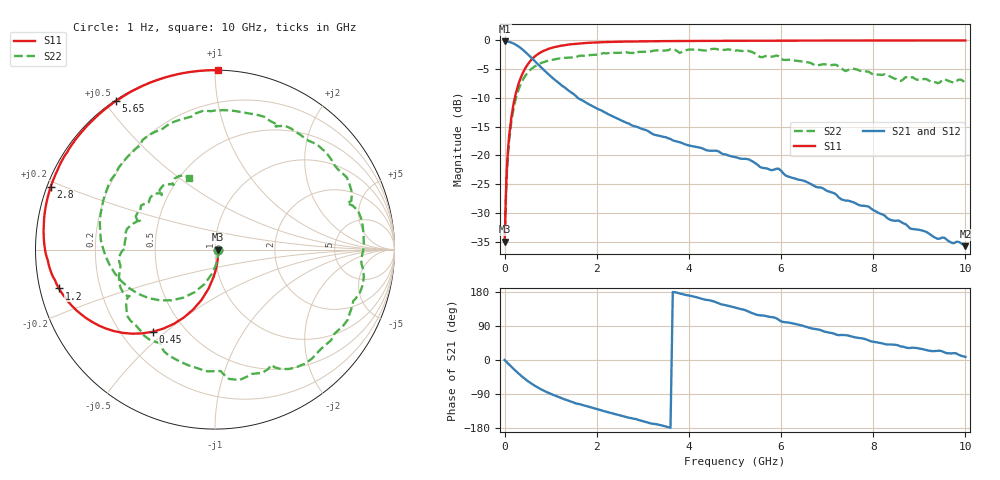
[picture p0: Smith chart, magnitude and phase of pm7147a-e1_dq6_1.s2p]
# GHz S DB R 50
! S-Parameters data
! Freq  dbS11  angS11  dbS21  angS21  dbS12  angS12  dbS22  angS22
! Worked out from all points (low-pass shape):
!   279 points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, 1 Hz to 10 GHz, reference 50 ohm
!   highest |S21| = -0.16 dB at 316.2 Hz (marker M1); lowest = -35.8 dB at 10 GHz (marker M2)
!   |S21| within 3 dB of the highest: start of sweep to 599.2 MHz
!   lowest |S11| = -35.0 dB at 316.2 Hz (marker M3), VSWR 1.04, Z = 51.8 - j4.22e-05 ohm
!   |S11| at or under -10 dB: start of sweep to 221.7 MHz
!   |S22| runs from -35.0 to -1.4 dB; largest |S21 - S12| = 3.9e-14
!   S11 on the Smith chart (normalised r, x): 1 Hz: 1.04, -0.00; 450 MHz: 0.33, -0.45; 1.2 GHz: 0.06, -0.12; 2.8 GHz: 0.01, +0.18; 5.65 GHz: 0.00, +0.54; 10 GHz: 0.00, +1.02
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1e-09  -35.00 -0.0  -0.16 -0.0  -0.16 -0.0  -35.00 -0.0
3.162e-07  -35.00 -0.0  -0.16 -0.0  -0.16 -0.0  -35.00 -0.0
0.03162278  -25.91 -71.9  -0.17 -3.9  -0.17 -3.9  -26.57 -71.9
0.06309573  -20.36 -85.0  -0.20 -7.7  -0.20 -7.7  -21.11 -87.4
0.15  -13.12 -99.4  -0.38 -18.2  -0.38 -18.2  -13.92 -107.1
0.3  -7.61 -114.6  -1.03 -35.3  -1.03 -35.3  -8.61 -130.4
0.45  -4.82 -127.2  -2.01 -50.7  -2.01 -50.7  -6.13 -150.0
0.8  -2.00 -149.5  -4.75 -77.9  -4.75 -77.9  -3.90 175.1
1.2  -0.95 -166.0  -7.56 -99.2  -7.56 -99.2  -3.13 145.8
1.7  -0.47 -179.9  -10.49 -119.0  -10.49 -119.0  -2.66 117.0
2.15  -0.30 170.5  -12.40 -134.7  -12.40 -134.7  -2.19 94.6
2.8  -0.17 159.1  -14.88 -155.1  -14.88 -155.1  -2.18 63.1
3.35  -0.12 151.0  -16.58 -170.8  -16.58 -170.8  -1.71 39.9
4.2  -0.08 139.7  -18.58 164.4  -18.58 164.4  -1.62 2.2
4.55  -0.07 135.6  -19.19 154.3  -19.19 154.3  -1.45 -13.4
5.05  -0.06 129.9  -20.38 136.7  -20.38 136.7  -1.72 -38.0
5.65  -0.04 123.6  -22.22 116.7  -22.22 116.7  -2.75 -66.0
5.95  -0.04 120.6  -22.32 106.1  -22.32 106.1  -2.79 -83.7
6.7  -0.02 113.6  -25.24 82.5  -25.24 82.5  -4.17 -119.0
7.6  -0.01 106.0  -28.25 59.9  -28.25 59.9  -4.97 -160.7
8.35  -0.01 100.2  -31.14 41.0  -31.14 41.0  -6.20 164.3
10  -0.00 89.1  -35.79 8.1  -35.79 8.1  -7.44 109.8
